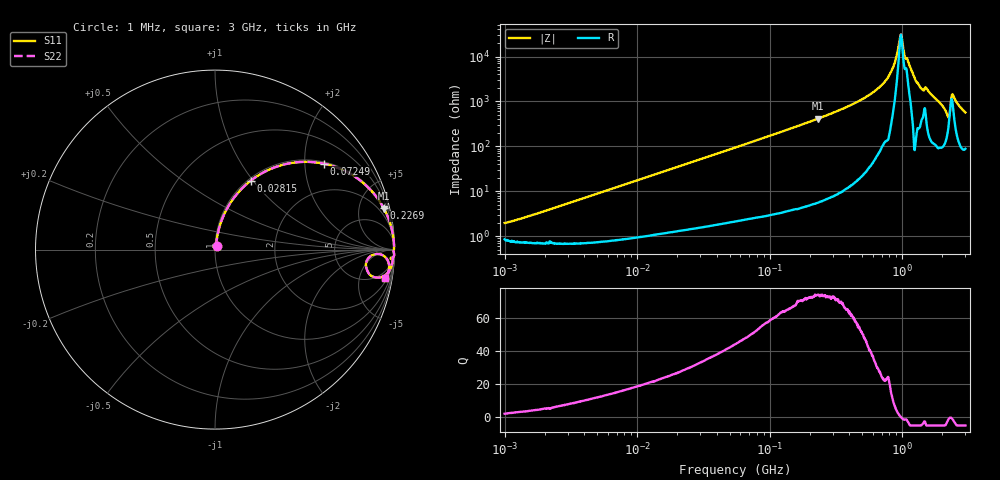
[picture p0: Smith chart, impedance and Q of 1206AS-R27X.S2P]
!s-Parameter Generated by FASTRON Sdn. Bhd.
!FASTRON P/N : 1206AS-R27X
!Keysight Technologies: E4991B_MY54100416_A.01.15
!Date created: Thu Nov 16 10:51:47 2023
!Version  : Rev00 Thu Nov 16 10:51:47 2023
!Data & Calibration Information:
!Freq	S11	S21	S12	S22
!PortZ  Port1:50+j0  Port2:50+j0
!When reading reference impedance value at option line is always used.
! Remarks : This data is being provided solely for informational purposes.
# Hz S dB R 50
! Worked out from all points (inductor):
!   1601 points, 1 MHz to 3 GHz, reference 50 ohm
!   read as one part in series: L = 285 nH near 1.259 MHz
!   highest Q = 73.7 at 230.3 MHz (marker M1), where L = 285 nH
!   self-resonance near 978 MHz
!   S11 on the Smith chart (normalised r, x): 1 MHz: 1.02, +0.04; 28.15 MHz: 1.03, +0.97; 72.49 MHz: 1.05, +2.49; 226.9 MHz: 1.11, +8.11; 3 GHz: 3, -11
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1000000  -34.10 63.3  -0.08 -1.0  -0.08 -1.0  -34.10 63.3
3804036  -23.42 80.2  -0.08 -3.8  -0.08 -3.8  -23.42 80.2
1.447069e7  -12.29 73.4  -0.36 -14.0  -0.36 -14.0  -12.29 73.4
2.815302e7  -7.27 62.6  -1.03 -25.6  -1.03 -25.6  -7.27 62.6
5.477226e7  -3.37 46.0  -2.86 -42.7  -2.86 -42.7  -3.37 46.0
7.248696e7  -2.24 38.3  -4.16 -50.6  -4.16 -50.6  -2.24 38.3
2.083556e8  -0.34 15.1  -11.69 -74.1  -11.69 -74.1  -0.34 15.1
2.268557e8  -0.28 13.8  -12.44 -75.4  -12.44 -75.4  -0.28 13.8
2.302869e8  -0.27 13.6  -12.58 -75.6  -12.58 -75.6  -0.27 13.6
5.258324e8  -0.04 4.7  -21.81 -84.1  -21.81 -84.1  -0.04 4.7
6.753166e8  -0.02 2.7  -26.45 -85.2  -26.45 -85.2  -0.02 2.7
7.925923e8  -0.01 1.6  -31.32 -85.9  -31.32 -85.9  -0.01 1.6
8.71647e8  -0.02 0.8  -36.63 -81.6  -36.63 -81.6  -0.02 0.8
9.538021e8  -0.03 0.2  -46.83 -47.6  -46.83 -47.6  -0.03 0.2
9.779672e8  -0.03 0.0  -49.84 -5.5  -49.84 -5.5  -0.03 0.0
1.075512e9  -0.05 -0.5  -39.35 54.5  -39.35 54.5  -0.05 -0.5
1.255985e9  -0.01 -1.9  -29.72 86.1  -29.72 86.1  -0.01 -1.9
1.395152e9  -0.10 -2.9  -25.80 75.9  -25.80 75.9  -0.10 -2.9
1.542004e9  -0.08 -3.0  -25.49 78.7  -25.49 78.7  -0.08 -3.0
2.188818e9  -0.72 -9.8  -14.81 59.3  -14.81 59.3  -0.72 -9.8
2.431346e9  -0.32 -3.6  -22.94 58.3  -22.94 58.3  -0.32 -3.6
3e9  -0.35 -9.6  -15.49 71.5  -15.49 71.5  -0.35 -9.6
